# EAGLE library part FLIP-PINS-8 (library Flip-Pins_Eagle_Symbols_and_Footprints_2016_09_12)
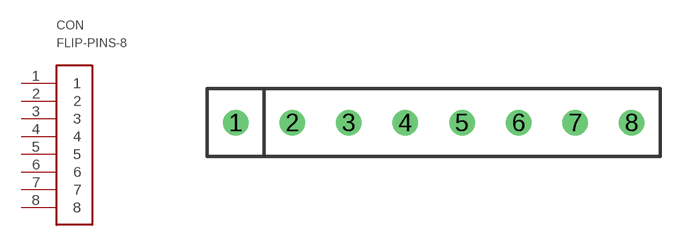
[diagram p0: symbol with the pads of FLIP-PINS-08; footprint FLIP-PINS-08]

Designator prefix CON

## FLIP-PINS-8  [FLIP-PINS-08]
1  1  pas
2  2  pas
3  3  pas
4  4  pas
5  5  pas
6  6  pas
7  7  pas
8  8  pas

## Footprint FLIP-PINS-08 (pad centres in mm)
drill 0.635 pad 1.016: 1 0,0; 2 2.54,0; 3 5.08,0; 4 7.62,0; 5 10.16,0; 6 12.7,0; 7 15.24,0; 8 17.78,0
